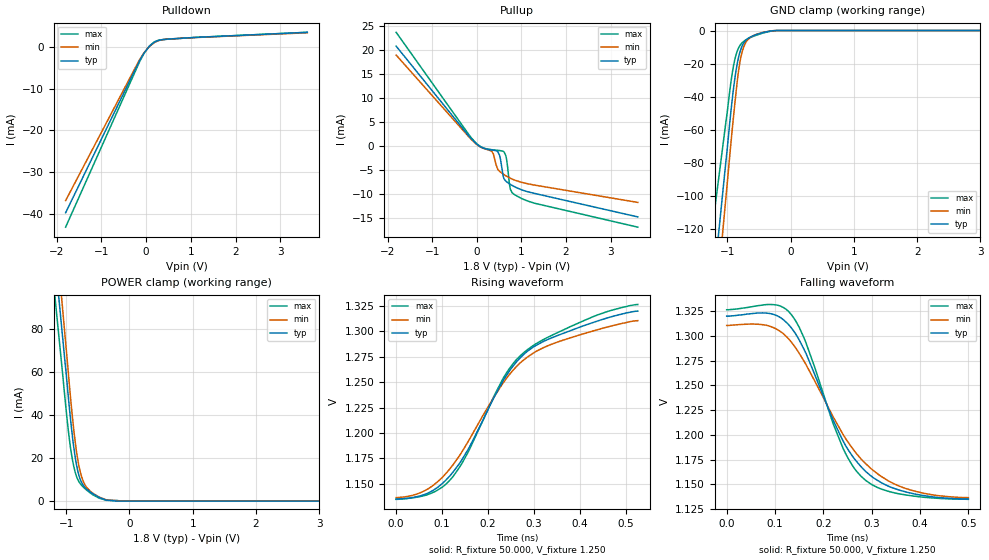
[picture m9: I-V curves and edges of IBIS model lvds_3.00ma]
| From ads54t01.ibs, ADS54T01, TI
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[Model]   lvds_3.00ma
Model_type 3-state
Vref=1.250E+00
Rref=5.000E+01
Cref=0.000E+00
Vmeas=1.250E+00
C_comp   7.860E-13   7.790E-13   7.930E-13
[Voltage Range]   1.800E+00   1.650E+00   1.950E+00
[POWER Clamp Reference]   1.800E+00   1.650E+00   1.950E+00
[GND Clamp Reference]   0.000E+00   0.000E+00   0.000E+00
[Pullup Reference]   1.800E+00   1.650E+00   1.950E+00
[Pulldown Reference]   0.000E+00   0.000E+00   0.000E+00
[Temperature Range]   25   85   -40
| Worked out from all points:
|   slope of the pulldown table from 0 to 0.27 V, typ, clamps not added: 115 ohm
|   slope of the pullup table from 0 to 0.27 V, typ, clamps not added: 245 ohm
|   GND clamp passes 1 mA (typ) near -0.41 V on its own axis
|   POWER clamp passes 1 mA (typ) near -0.41 V on its own axis
|   rising waveform, R_fixture 50.000, V_fixture 1.250: 20-80 % time 153ps typ, 161ps min, 159ps max; typ from 1.14 V to 1.32 V
|   falling waveform, R_fixture 50.000, V_fixture 1.250: 20-80 % time 107ps typ, 128ps min, 87.4ps max; typ from 1.32 V to 1.14 V
[GND Clamp]
-1.8V     -374.4mA   -423.5mA   -288.4mA
-1.02V    -78.69mA   -100.5mA   -54.92mA
-920mV    -41.17mA   -59.34mA   -25.51mA
-860mV    -23.88mA   -36.88mA   -14.48mA
-820mV    -15.94mA   -23.97mA   -10.43mA
-780mV    -10.76mA   -15.27mA   -8.038mA
-740mV    -7.589mA   -9.923mA   -6.562mA
-700mV    -5.657mA   -6.755mA   -5.499mA
-640mV    -4.069mA   -4.329mA   -4.359mA
-460mV    -1.489mA   -1.354mA   -1.806mA
-220mV    -4.201uA   -14.01uA   -11.29uA
3.6V      0A         0A         0A
[Power Clamp]
-1.8V     302.8mA    334.3mA    279.3mA
-1.76V    290.6mA    320.1mA    266.6mA
-1.06V    77.25mA    90.47mA    60.21mA
-940mV    40.5mA     50.88mA    26.54mA
-880mV    24.97mA    33.1mA     16.1mA
-820mV    14.43mA    19.78mA    10.24mA
-780mV    10.23mA    13.83mA    8.195mA
-720mV    6.913mA    8.542mA    6.262mA
-580mV    3.451mA    3.702mA    2.982mA
-360mV    441.4uA    538.8uA    356.5uA
-140mV    0A         9.789uA    18.55uA
3.6V      0A         0A         0A
[Pullup]
-1.81V    20.79mA    18.94mA    23.68mA
-30mV     573.8uA    485.1uA    689.4uA
330mV     -851.6uA   -1.075mA   -789.8uA
370mV     -901.1uA   -1.665mA   -836uA
470mV     -1.211mA   -4.92mA    -936.1uA
510mV     -1.966mA   -5.314mA   -976.1uA
610mV     -6.885mA   -5.994mA   -1.268mA
670mV     -7.516mA   -6.347mA   -2.973mA
730mV     -7.903mA   -6.654mA   -7.929mA
790mV     -8.246mA   -6.918mA   -9.773mA
1.29V     -9.909mA   -8.178mA   -11.95mA
3.61V     -14.82mA   -11.79mA   -16.96mA
[Pulldown]
-1.8V     -39.74mA   -36.82mA   -43.18mA
-140mV    -3.144mA   -2.933mA   -3.403mA
-40mV     -1.365mA   -1.299mA   -1.444mA
60mV      757.4nA    -39.41uA   57.93uA
180mV     1.107mA    1.018mA    1.2mA
340mV     1.712mA    1.68mA     1.715mA
540mV     1.918mA    1.921mA    1.886mA
3.6V      3.501mA    3.395mA    3.501mA
[Rising Waveform]
R_fixture = 50.000
V_fixture = 1.250
V_fixture_min = 1.250
V_fixture_max = 1.250
|  time   V(typ)   V(min)   V(max)
0s        1.135V     1.137V     1.135V
68ps      1.141V     1.145V     1.139V
120ps     1.159V     1.167V     1.155V
156ps     1.183V     1.191V     1.181V
234ps     1.252V     1.25V      1.255V
260ps     1.269V     1.264V     1.271V
286ps     1.281V     1.275V     1.282V
336ps     1.293V     1.287V     1.296V
428ps     1.309V     1.3V       1.314V
526ps     1.32V      1.311V     1.327V
[Falling Waveform]
R_fixture = 50.000
V_fixture = 1.250
V_fixture_min = 1.250
V_fixture_max = 1.250
|  time   V(typ)   V(min)   V(max)
0s        1.32V      1.311V     1.327V
88ps      1.323V     1.31V      1.332V
134ps     1.308V     1.294V     1.321V
164ps     1.282V     1.271V     1.293V
220ps     1.215V     1.218V     1.212V
242ps     1.193V     1.199V     1.185V
264ps     1.176V     1.184V     1.166V
288ps     1.163V     1.171V     1.154V
370ps     1.142V     1.146V     1.139V
500ps     1.135V     1.137V     1.135V
[Ramp]
dV/dt_r   1.1094E-01/1.5250E-10   1.0446E-01/1.6090E-10   1.1502E-01/1.5850E-10
dV/dt_f   1.1094E-01/1.0691E-10   1.0446E-01/1.2806E-10   1.1502E-01/8.7078E-11
R_load = 50
